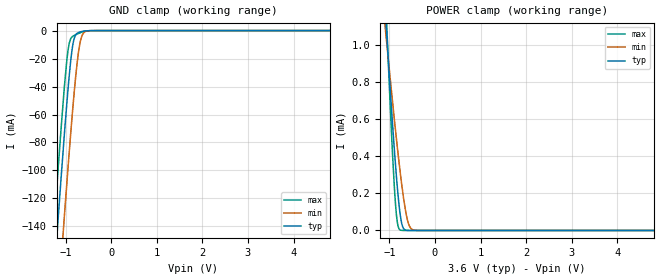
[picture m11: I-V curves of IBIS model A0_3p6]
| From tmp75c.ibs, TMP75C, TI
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|   Model
[Model]   A0_3p6
Model_type   Input
Vinl = 0.9
Vinh = 2.1
|   typ   min   max
C_comp   0.383pF   0.370pF   0.391pF
[Voltage Range]   3.6   3.59   3.61
[Temperature Range]   25   125   -40
[Power Clamp Reference]   3.6   3.59   3.61
[GND Clamp Reference]   0   0   0
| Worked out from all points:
|   GND clamp passes 1 mA (typ) near -0.68 V on its own axis
|   POWER clamp passes 1 mA (typ) near -1.04 V on its own axis
[GND Clamp]
|   Voltage   I(typ)   I(min)   I(max)
-3.6V     -1.323A    -1.379A    -1.29A
-1.278V   -187mA     -247.1mA   -151mA
-1.192V   -147mA     -207mA     -111mA
-1.181V   -142mA     -202mA     -106.1mA
-1.094V   -103mA     -162.6mA   -67.73mA
-1.03V    -74.89mA   -133.6mA   -40.99mA
-943.2mV  -40.15mA   -96.06mA   -13.07mA
-835.2mV  -8.827mA   -52.55mA   -3.897mA
-716.4mV  -1.383mA   -15.13mA   -2.039mA
-619.2mV  -502.6uA   -2.225mA   -893uA
-478.8mV  -65.17uA   -114.9uA   -103.9uA
7.2V      0A         0A         0A
[POWER Clamp]
|   Voltage   I(typ)   I(min)   I(max)
-3.6V     12.4mA     8.145mA    18.7mA
-1.105V   1.239mA    1.127mA    1.392mA
-1.051V   1.024mA    989.3uA    1.066mA
-975.6mV  734.6uA    800.6uA    636.7uA
-889.2mV  428.3uA    592.9uA    225.3uA
-824.4mV  229.1uA    445uA      42.14uA
-759.6mV  80.08uA    307.1uA    2.394uA
-705.6mV  18.42uA    203.3uA    159.6nA
-608.4mV  508.2nA    61.2uA     0A
-532.8mV  20.23nA    12.14uA    0A
-435.6mV  0A         832.8nA    0A
7.2V      0A         0A         0A
